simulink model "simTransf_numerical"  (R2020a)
settings: Solver=ode15s  StartTime=0.0  StopTime=tsim  FixedStep=0.1  MaxStep=1  RelTol=1e-5
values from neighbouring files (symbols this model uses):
  C = m.c*cp.c/(m.h*cp.h)    [eNTU.m]    (also in runTransf.m = [zeros(1,2*N-1),1]; calcblock.m = Fc*cpc/(Fh*cph); Main.m = [zeros(1,2*N-1),1]; Main_OL.m = [zeros(1,2*N-1),1])
  d_tstep = [500 5000 7000 13000]    [runTransf.m]    (also in Main.m = [1000; 1000;2000]; Main_OL.m = 300; runTestCalcBlk.m = 300; runTransfOL.m)
  dFfeed = 0    [runTransf.m]
  dFh = 0    [runTransf.m]    (also in Main.m = 0;0.2*Fh; runTransfOL.m)
  dm = 0    [runTransf.m]
  dTcin = 0    [runTransf.m]    (also in Main.m = 2; runTransfOL.m)
  dTfeed = 0    [runTransf.m]
  dU = 0    [runTransf.m]    (also in runTransfOL.m)
  dvsp = [5;5];vsp0*0    [runTransf.m]    (also in runTransfOL.m = [0;0];vsp0*0)
  Fc0 = 5    [runTransf.m]    (also in Main.m; Main_OL.m; runTestCalcBlk.m; runTransfOL.m)
  Ffeed0 = (1-R)/R*Fh    (= 27)    [runTransf.m]
  Fh = d(1)    [calcblk.m]    (also in calcv.m; calcv0w.m; runTransf.m = 3; TankWithHEXode.m)
  KI = 1/kS(i)*1/tauCS(i)    [runTransf.m]    (also in Main.m = Kp/tauIv; Main_OL.m = 1; runTransfOL.m)
  Kp = 1    [runTransf.m]    (also in Main.m = 1/kv*tauv/(tauC+thetav); Main_OL.m = 0)
  m0 = taur*Ffeed0    (= 48600)    [runTransf.m]
  nd = size(d0,2)    [runTransf.m]    (also in Main.m; Main_OL.m; runTestCalcBlk.m; runTransfOL.m)
  np = size(p,2)    [runTransf.m]    (also in runH2Psim.m = length(param); Main.m; Main_OL.m; runTestCalcBlk.m)
  nu = 1    [runTransf.m]    (also in runH2Psim.m = length(u0); Main.m; Main_OL.m; runTestCalcBlk.m)
  nx = size(x0,1)    [runTransf.m]    (also in H2P_Turbine_driven.m = param(end); runTD.m = length(x0); H2P_Boiler_driven.m = param(end); runBD.m = length(x0))
  OLorCL = 1    [runTransf.m]
  p = [N, Fc0, rhoc, rhoh, U0, A,cpc,cph]    [runTransf.m]    (also in Main.m = [N, Fc0, rhoc, rhoh,U,A,cpc,cph]; Main_OL.m = [N, Fc0, rhoc, rhoh,U,A,cpc,cph]; runTestCalcBlk.m = [N, Fc0, rhoc, rhoh,U,A,cpc,cph]; NonlinearMap.m = [U;A;Fc(i);Fh;cpc;cph;Tcin;Thin])
  Tcin = d(2)    [calcblk.m]    (also in calcv.m; calcv0.m; calcv0w.m; calcvE.m)
  Tfeed0 = Fh/Ffeed0*(Thin-Thend(N)) + Thin    [runTransf.m]
  Thsp = Thsp0    [runTransf.m]    (also in Main.m = Thsp0+dThsp; Main_OL.m = Thsp0+dThsp; runTestCalcBlk.m = Thsp0+dThsp; runTransfOL.m)
  Thsp0 = x0(end);  2.971202611676064e+02    [runTransf.m]    (also in Main.m = Thend(end); Main_OL.m = 297.120261168; runTestCalcBlk.m = Thend(end); runTransfOL.m)
  trf = zeros(3,1)    [runTransf.m]    (also in runTransfOL.m)
  tstep = 10000    [runTransf.m]    (also in Main_OL.m = 100; Main.m = 100; runTransfOL.m = 100)
  U0 = 150    [runTransf.m]    (also in runTransfOL.m)
  v0 = 0    [runTransf.m]    (also in runTD.m = v(end,:); runBD.m = v(end,:); runFP.m = v(end,:); runFPV2.m = v(end,:))
  vf = 0    [runTransf.m]    (also in Main.m = v0+dThsp; runTransfOL.m = v00)
  vsp0 = [v00; Thin + (Fc0* cpc)/(Fh*cph)*(Tcin-x0(1)); Fc0*(Tcin-x0(1))]    [runTransf.m]    (also in runTransfOL.m)
  x0 = [Tcend(1:N)'; Thend(1:N)']    [runTransf.m]    (also in runTD.m = [TE0;TD0;TSh0;MD0; MSh0;w0;TA0;0;0;0;0;0;0;0;0;0]; runBD.m = [TE0;TD0;TSh0;MD0; MSh0;w0;TA0;0;0;0;0;0;0;0;0;0]; runFP.m = [TE0;TD0;TSh0;MD0; MSh0;w0;TA0;0;0;0;0;0;0;0]; runFPV2.m = [TE0;TD0;TSh0;MD0; MSh0;w0;TA0;0;0;0;0;0;0;0])
undefined symbols (not defined in the file or in its folder): TankWithHEXode

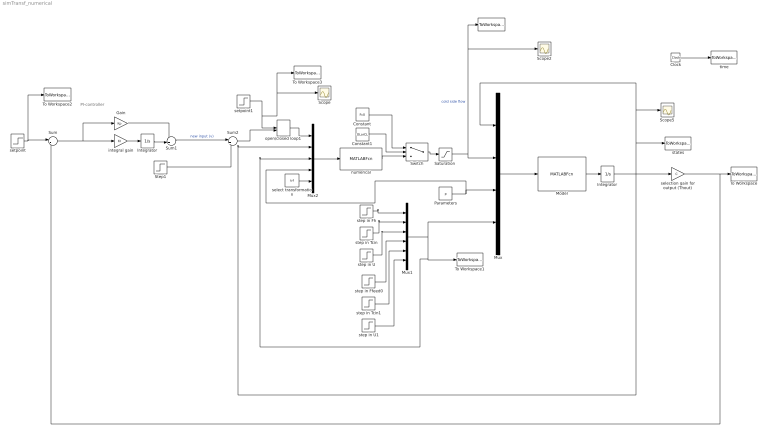
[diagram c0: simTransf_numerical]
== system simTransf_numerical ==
  note: PI-controller
  " " : ToWorkspace  VariableName=u  SampleTime=-1
  Clock : Clock
  Constant : Constant  Value=Fc0
  Constant1 : Constant  Value=OLorCL
  Gain : Gain  Gain=Kp
  Integrator : Integrator
  "Integrator " : Integrator  InitialCondition=x0
  Model : MATLABFcn  MATLABFcn=TankWithHEXode(u(1:nx),u(nx+1:nx+nu),u(nx+nu+1:nx+nu+np),u(nx+nu+np+1:nx+nu+np+nd))  OutputDimensions=nx  Output1D=off
  Mux : Mux
  Mux1 : Mux  Inputs=6
  Mux2 : Mux  Inputs=5
  Parameters : Constant  Value=p
  "Saturation " : Saturate  UpperLimit=10  LowerLimit=0
  Scope : Scope
  Scope2 : Scope
  Scope5 : Scope
  Step1 : Step  Time=tstep  Before=v0  After=vf  SampleTime=0
  Sum : Sum  Inputs=|+-
  Sum1 : Sum  Inputs=++|
  Sum2 : Sum  Inputs=|++
  Switch : Switch  Criteria=u2 > Threshold
  To Workspace : ToWorkspace  VariableName=Thout  SampleTime=-1
  To Workspace1 : ToWorkspace  VariableName=dsim  SampleTime=-1
  To Workspace2 : ToWorkspace  VariableName=Tsp  SampleTime=-1
  To Workspace3 : ToWorkspace  VariableName=ysp  SampleTime=-1
  integral gain : Gain  Gain=KI  Multiplication=Matrix(K*u)
  numerical : MATLABFcn  MATLABFcn=calcblk(u(1),u(2:nx+1),u(nx+2:nx+nd+1),u(nx+nd+2:nx+nd+np+1),u(end))
  open/closed loop1 : ManualSwitch
  select transformation : Constant  Value=trf
  selection gain for output (Thout) : Gain  Gain=C  Multiplication=Matrix(K*u)
  setpoint : Step  Time=tstep  Before=Thsp0  After=Thsp  SampleTime=0
  setpoint1 : Step  Time=tstep  Before=vsp0  After=vsp0+dvsp  SampleTime=0
  states : ToWorkspace  VariableName=y  SampleTime=-1
  step in Ffeed0 : Step  Time=d_tstep(4)  Before=Ffeed0  After=Ffeed0 + dFfeed  SampleTime=0
  step in Fh : Step  Time=d_tstep(1)  Before=Fh  After=Fh+dFh  SampleTime=0
  step in Tcin : Step  Time=d_tstep(2)  Before=Tcin  After=Tcin+dTcin  SampleTime=0
  step in Tcin1 : Step  Time=d_tstep(5)  Before=m0  After=m0+dm  SampleTime=0
  step in U : Step  Time=d_tstep(3)  Before=U0  After=U0-dU  SampleTime=0
  step in U1 : Step  Time=d_tstep(6)  Before=Tfeed0  After=Tfeed0+dTfeed  SampleTime=0
  time : ToWorkspace  VariableName=t  SampleTime=-1
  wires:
  Model/1 -> "Integrator "/1
  "Integrator "/1 -> Mux2/2, selection gain for output (Thout)/1, states/1, Mux/1, Scope5/1
  Mux/1 -> Model/1
  Clock/1 -> time/1
  Parameters/1 -> Mux2/4, Mux/3
  "Saturation "/1 -> Mux/2, Scope2/1, " "/1  "cold side flow"
  numerical/1 -> Switch/3
  setpoint/1 -> To Workspace2/1, Sum/1
  Sum/1 -> Gain/1, integral gain/1
  integral gain/1 -> Integrator/1
  Sum1/1 -> Sum2/1  "new input (v)"
  selection gain for output (Thout)/1 -> Sum/2, To Workspace/1
  Mux2/1 -> numerical/1
  Step1/1 -> Sum2/2
  Switch/1 -> "Saturation "/1
  Constant/1 -> Switch/1
  Integrator/1 -> Sum1/2
  open/closed loop1/1 -> Mux2/1
  setpoint1/1 -> Scope/1, To Workspace3/1, open/closed loop1/1
  Gain/1 -> Sum1/1
  Sum2/1 -> open/closed loop1/2
  select transformation/1 -> Mux2/5
  step in U1/1 -> Mux1/6
  step in Ffeed0/1 -> Mux1/4
  step in Tcin1/1 -> Mux1/5
  step in Fh/1 -> Mux1/1
  Mux1/1 -> Mux2/3, To Workspace1/1, Mux/4
  step in U/1 -> Mux1/3
  step in Tcin/1 -> Mux1/2
  Constant1/1 -> Switch/2
